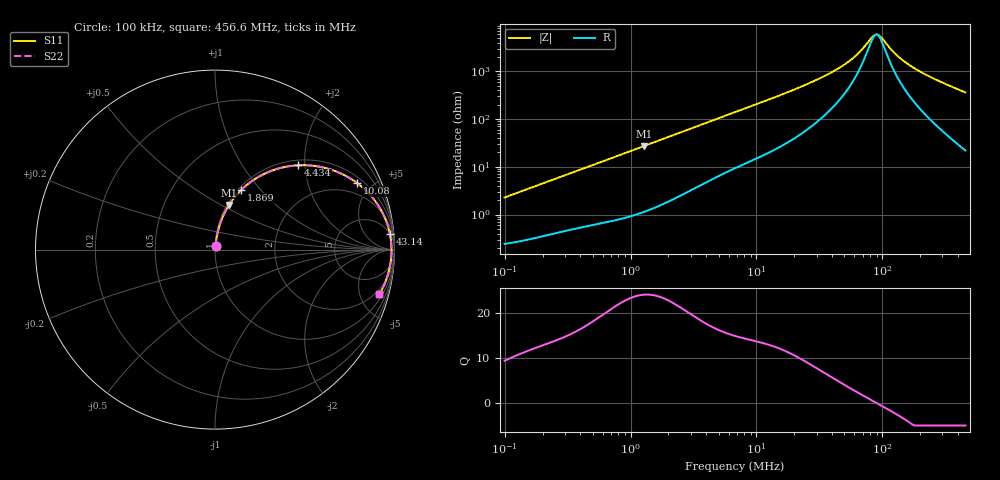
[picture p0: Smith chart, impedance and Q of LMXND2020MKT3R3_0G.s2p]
! LMXND2020MKT3R3_0G  S-PARAMETER MODEL  ( General Type )
! Model Generated by TAIYO YUDEN Corporation (https://www.yuden.co.jp/en/)
! Version 1.0
! TAIYO YUDEN Control No. 191023NI43SB-FBB
! Copyright(c) 2019 TAIYO YUDEN CO.,LTD. All Rights Reserved.
! Product Description (link to TY-COMPAS)
! https://ds.yuden.co.jp/TYCOMPAS/or/detail?pn=LMXND2020MKT3R3M0G&u=M
! Products Name : Inductors
! Characteristics :
!  Inductance : 3.3 uH , SRF(min) : -Hz , DC Resistance(max) : 0.228 Ohm
!  Rated Current : Saturation :1000 mA , Temp Rise : 1020 mA (40 degC)
!  Case Size : 2.0 x 2.0 / 0.079 x 0.079 [mm/inch] , Thickness : 1.2 / 0.047 [mm/inch]
!  (Conditions: Temperature = 25 degC , DC Bias Current/Voltage = 0A / 0V)
! External Node Assignments :
!  1  o---GGG---o  2
! GND o---------o GND
! Frequency Range : 0.1MHz  -  456.598367MHz  [ 402 STEP ]
# MHz S RI R 50
! Freq[MHz].  S11 Real  S11 Imag  S21 Real  S21 Imag  S12 Real  S12 Imag  S22 Real  S22 Imag
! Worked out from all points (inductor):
!   401 points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, 100 kHz to 456.6 MHz, reference 50 ohm
!   read as one part in series: L = 3.59 uH near 104.3 kHz
!   highest Q = 24 at 1.279 MHz (marker M1), where L = 3.39 uH
!   self-resonance near 89.88 MHz
!   S11 on the Smith chart (normalised r, x): 100 kHz: 1.00, +0.05; 1.869 MHz: 1.03, +0.79; 4.434 MHz: 1.11, +1.84; 10.08 MHz: 1.30, +4.10; 43.14 MHz: 5, +21; 456.6 MHz: 1.44, -7.23
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0.1  0.00294 0.0226  0.9971 -0.0226  0.9971 -0.0226  0.00294 0.0226
0.410178  0.0132 0.0877  0.9868 -0.0877  0.9868 -0.0877  0.0132 0.0877
0.739843  0.0316 0.1528  0.9684 -0.1528  0.9684 -0.1528  0.0316 0.1528
1.279408  0.0783 0.2486  0.9217 -0.2486  0.9217 -0.2486  0.0783 0.2486
1.682457  0.1236 0.3086  0.8764 -0.3086  0.8764 -0.3086  0.1236 0.3086
1.86934  0.1467 0.3327  0.8533 -0.3327  0.8533 -0.3327  0.1467 0.3327
2.789434  0.2671 0.4184  0.7329 -0.4184  0.7329 -0.4184  0.2671 0.4184
4.433947  0.4625 0.4698  0.5375 -0.4698  0.5375 -0.4698  0.4625 0.4698
6.901063  0.6575 0.4418  0.3425 -0.4418  0.3425 -0.4418  0.6575 0.4418
10.08312  0.7916 0.371  0.2084 -0.371  0.2084 -0.371  0.7916 0.371
16.02764  0.8966 0.265  0.1034 -0.265  0.1034 -0.265  0.8966 0.265
27.71655  0.9554 0.1546  0.0446 -0.1546  0.0446 -0.1546  0.9554 0.1546
43.13847  0.9746 0.0865  0.0254 -0.0865  0.0254 -0.0865  0.9746 0.0865
60.4291  0.981 0.0443  0.019 -0.0443  0.019 -0.0443  0.981 0.0443
82.88552  0.9832 0.00885  0.0168 -0.00885  0.0168 -0.00885  0.9832 0.00885
88.29277  0.9834 0.00194  0.0166 -0.00194  0.0166 -0.00194  0.9834 0.00194
96.05512  0.9834 -0.00726  0.0166 0.00726  0.0166 0.00726  0.9834 -0.00726
113.6871  0.9828 -0.0259  0.0172 0.0259  0.0172 0.0259  0.9828 -0.0259
140.3458  0.981 -0.0502  0.019 0.0502  0.019 0.0502  0.981 -0.0502
188.4878  0.9757 -0.0878  0.0243 0.0878  0.0243 0.0878  0.9757 -0.0878
281.262  0.9602 -0.1499  0.0398 0.1499  0.0398 0.1499  0.9602 -0.1499
456.5984  0.9161 -0.2485  0.0839 0.2485  0.0839 0.2485  0.9161 -0.2485
